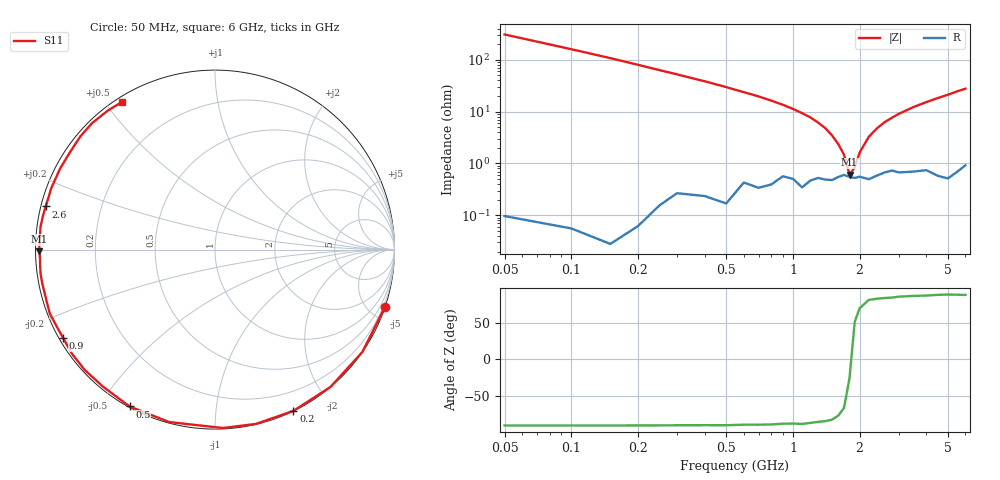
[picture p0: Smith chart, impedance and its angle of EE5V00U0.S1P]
! Infineon Technologies  Discrete & RF Semiconductors
! BBY55-02W
! Si Tuning Diode in SCD-80
! VR = 5 V
! S-Parameters:  June  2000
# GHz  S  MA  R  50
!  f  S11
! GHz  MAG  ANG
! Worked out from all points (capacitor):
!   34 points, 50 MHz to 6 GHz, reference 50 ohm
!   read as one part to ground: C = 9.95 pF near 50 MHz
!   lowest |Z| = 610 mohm at 1.8 GHz (marker M1)
!   series resonance near 1.829 GHz, so ESL is about 760 pH
!   S11 on the Smith chart (normalised r, x): 50 MHz: 0.00, -6.14; 200 MHz: 0.00, -1.60; 500 MHz: 0.00, -0.59; 900 MHz: 0.01, -0.27; 2.6 GHz: 0.01, +0.13; 6 GHz: 0.02, +0.55
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0.05  0.9999 -18.5
0.1  0.9998 -34.8
0.15  0.9998 -49.9
0.2  0.9993 -64.1
0.25  0.9976 -76.8
0.3  0.9949 -87.5
0.4  0.9941 -104.9
0.5  0.995 -118.6
0.6  0.9861 -129.2
0.7  0.9883 -137.2
0.8  0.9858 -144.0
0.9  0.9791 -149.7
1  0.9809 -154.6
1.1  0.9867 -158.9
1.3  0.9795 -166.1
1.5  0.9811 -172.1
1.6  0.9784 -174.7
1.8  0.9782 -179.4
2.2  0.9804 172.6
2.4  0.977 169.1
2.6  0.9738 165.7
3  0.9743 159.6
3.5  0.974 152.5
4  0.9732 146.1
4.5  0.9798 139.9
5  0.9827 134.2
5.5  0.9781 127.8
6  0.9722 122.1
